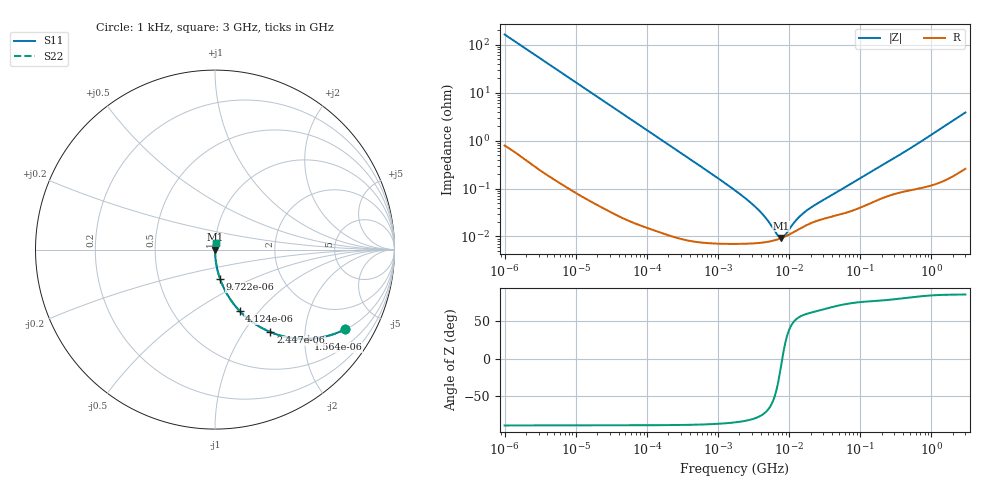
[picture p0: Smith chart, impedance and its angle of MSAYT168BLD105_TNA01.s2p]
! MSAYT168BLD105_TNA01  S-PARAMETER MODEL  ( Standard Model )
! Model Generated by TAIYO YUDEN Corporation (http://www.ty-top.com)
! Version 1.0
! TAIYO YUDEN Control No. 220601
! Copyright(c) 2012 TAIYO YUDEN CO.,LTD. All Rights Reserved.
! Product Description (link to TY-COMPAS)
! https://ds.yuden.co.jp/TYCOMPAS/or/detail?pn=MSAYT168BLD105KTNA01&u=M
! Products Name : Multilayer Ceramic Capacitors
! Characteristics :
!  Capacitance : 1 [uF] , Rated Voltage : 25 [V] , TCC : X5R
!  Case Size : 1.6 x 0.8 / 0.063 x 0.031 [mm/inch] , Thickness : 0.8 / 0.031 [mm/inch]
!  (Conditions: Temperature = 25 [degC] , DC Bias Voltage = 0 [V])
! External Node Assignments :
!  1  o---| |---o  2
! GND o---------o GND
! Frequency Range : 1kHz  -  3GHz  [ 401 STEP ]
# MHZ S RI R 50
! Freq[MHz].  S11 Real  S11 Imag  S21 Real  S21 Imag  S12 Real  S12 Imag  S22 Real  S22 Imag
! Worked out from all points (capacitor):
!   401 points, 1 kHz to 3 GHz, reference 50 ohm
!   read as one part in series: C = 977 nF near 1.077 kHz
!   lowest |Z| = 9.34 mohm at 7.696 MHz (marker M1)
!   series resonance near 8.001 MHz, so ESL is about 400 pH
!   S11 on the Smith chart (normalised r, x): 1 kHz: 1.02, -3.25; 1.564 kHz: 1.01, -2.08; 2.447 kHz: 1.01, -1.33; 4.124 kHz: 1.00, -0.79; 9.722 kHz: 1.00, -0.34; 3 GHz: 1.01, +0.08
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0.001  0.7247 -0.4442  0.2753 0.4442  0.2753 0.4442  0.7247 -0.4442
0.001564  0.5203 -0.4972  0.4797 0.4972  0.4797 0.4972  0.5203 -0.4972
0.002447  0.3086 -0.4596  0.6914 0.4596  0.6914 0.4596  0.3086 -0.4596
0.004124  0.1368 -0.3414  0.8632 0.3414  0.8632 0.3414  0.1368 -0.3414
0.005988  0.0705 -0.2536  0.9295 0.2536  0.9295 0.2536  0.0705 -0.2536
0.009722  0.0284 -0.1635  0.9716 0.1635  0.9716 0.1635  0.0284 -0.1635
0.01216  0.0185 -0.1322  0.9815 0.1322  0.9815 0.1322  0.0185 -0.1322
0.033275  0.00274 -0.0492  0.9973 0.0492  0.9973 0.0492  0.00274 -0.0492
0.147855  0.000248 -0.0112  0.9998 0.0112  0.9998 0.0112  0.000248 -0.0112
1.732051  7.08e-05 -0.000913  0.9999 0.000913  0.9999 0.000913  7.08e-05 -0.000913
2.610246  7.11e-05 -0.000567  0.9999 0.000567  0.9999 0.000567  7.11e-05 -0.000567
3.651041  7.31e-05 -0.000359  0.9999 0.000359  0.9999 0.000359  7.31e-05 -0.000359
4.919932  7.71e-05 -0.000208  0.9999 0.000208  0.9999 0.000208  7.71e-05 -0.000208
6.629817  8.53e-05 -7.71e-05  0.9999 7.71e-05  0.9999 7.71e-05  8.53e-05 -7.71e-05
7.143107  8.84e-05 -4.61e-05  0.9999 4.61e-05  0.9999 4.61e-05  8.84e-05 -4.61e-05
7.696136  9.21e-05 -1.57e-05  0.9999 1.57e-05  0.9999 1.57e-05  9.21e-05 -1.57e-05
8.933959  0.000101 4.4e-05  0.9999 -4.4e-05  0.9999 -4.4e-05  0.000101 4.4e-05
11.59828  0.000124 0.000145  0.9999 -0.000145  0.9999 -0.000145  0.000124 0.000145
13.97519  0.000144 0.000215  0.9999 -0.000215  0.9999 -0.000215  0.000144 0.000215
21.06097  0.000194 0.00037  0.9998 -0.00037  0.9998 -0.00037  0.000194 0.00037
256.0921  0.000724 0.00368  0.9993 -0.00368  0.9993 -0.00368  0.000724 0.00368
3000  0.00403 0.0381  0.996 -0.0381  0.996 -0.0381  0.00403 0.0381
